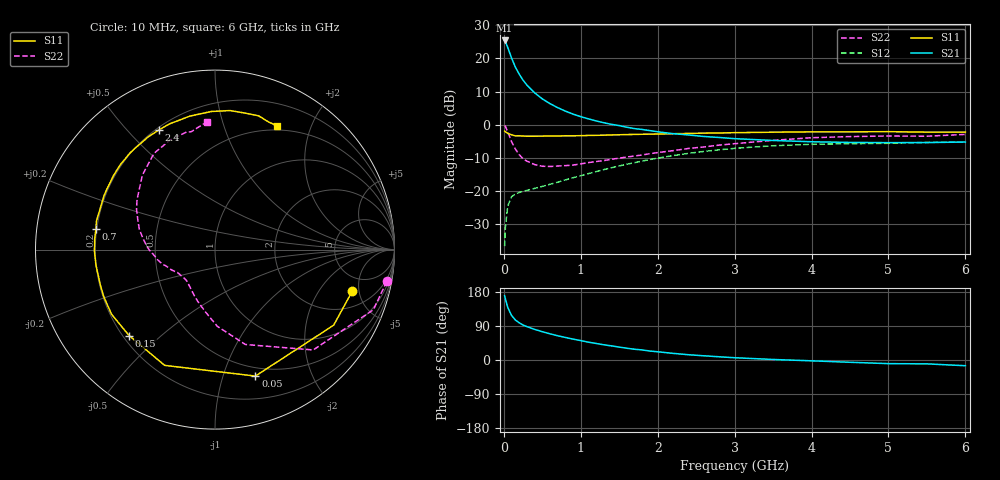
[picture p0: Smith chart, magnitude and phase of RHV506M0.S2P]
! SIEMENS Small Signal Semiconductors
! BFR106
! Si NPN RF Bipolar Junction Transistor in SOT23
! VCE = 0.5 V  IC = 6 mA
! Common Emitter S-Parameters:  August  1996
# GHz  S  MA  R  50
!  f  S11  S21  S12  S22
! GHz  MAG  ANG  MAG  ANG  MAG  ANG  MAG  ANG
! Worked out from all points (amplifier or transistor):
!   36 points, 10 MHz to 6 GHz, reference 50 ohm
!   highest |S21| = 25.4 dB at 10 MHz (marker M1)
!   |S21| within 3 dB of that: start of sweep to 64.42 MHz
!   unconditionally stable (mu >= 1): 527.6 MHz to end of sweep
!   at 250 MHz: K = 0.59, MSG = 16.8 dB, |S12| = -20.2 dB
!   at 1.4 GHz: K = 1.19, MAG = 3.9 dB, |S12| = -13.0 dB
!   at 6 GHz: K = 1.03, MAG = -1.1 dB, |S12| = -5.1 dB
!   S11 on the Smith chart (normalised r, x): 10 MHz: 3.30, -4.25; 50 MHz: 0.41, -1.28; 150 MHz: 0.22, -0.40; 700 MHz: 0.20, +0.08; 2.4 GHz: 0.21, +0.62; 6 GHz: 0.45, +1.53
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0.01  0.799 -16.9  18.72 169.8  0.0146 82.1  0.9733 -10.5
0.02  0.7839 -32.5  17.99 161.6  0.0281 75.1  0.9439 -20.8
0.05  0.7397 -72.3  14.73 139.1  0.0587 55.1  0.7825 -45.6
0.1  0.7034 -113.5  10.2 117.7  0.0814 39.6  0.5553 -72.2
0.15  0.6771 -135.0  7.392 105.5  0.0899 33.2  0.4274 -88.3
0.2  0.6796 -148.0  5.794 98.1  0.0946 31.1  0.3525 -98.5
0.25  0.673 -156.9  4.695 92.2  0.0982 30.7  0.3054 -108.1
0.3  0.6685 -162.9  3.961 88.1  0.1018 31.4  0.2813 -114.2
0.4  0.6689 -172.7  3.031 80.8  0.1089 33.6  0.2495 -124.4
0.5  0.6716 -179.1  2.453 74.7  0.1167 36.4  0.2353 -131.7
0.6  0.673 175.1  2.078 69.1  0.1257 38.9  0.2335 -136.9
0.7  0.6732 170.2  1.808 64.0  0.1352 41.1  0.2372 -141.3
0.9  0.6784 162.4  1.443 55.1  0.1579 44.5  0.2452 -148.8
1.1  0.6873 154.1  1.224 47.0  0.1822 46.5  0.2674 -155.0
1.3  0.6935 147.3  1.069 40.1  0.2095 47.0  0.2866 -161.3
1.6  0.709 138.0  0.913 31.0  0.2526 46.3  0.3249 -170.0
2.2  0.7301 120.6  0.731 17.5  0.3408 39.9  0.4049 171.5
2.4  0.7366 115.0  0.699 13.9  0.369 36.8  0.4371 164.8
3.5  0.7698 91.5  0.577 1.4  0.4802 18.7  0.58 134.2
4.5  0.7789 77.4  0.539 -6.0  0.5159 3.8  0.6603 112.1
5.5  0.771 67.1  0.537 -10.2  0.5384 -4.8  0.6694 101.5
6  0.7717 63.4  0.546 -15.1  0.5531 -11.1  0.7122 93.8
